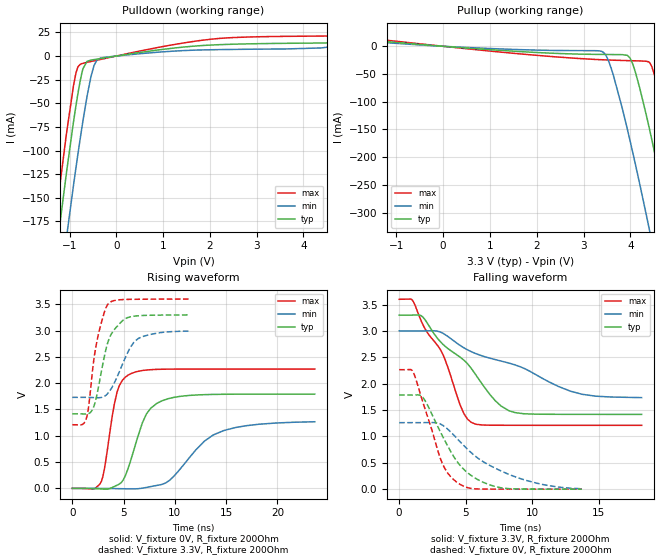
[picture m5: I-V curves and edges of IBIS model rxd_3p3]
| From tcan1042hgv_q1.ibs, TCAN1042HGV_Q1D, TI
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|   rxd_3p3 Model
[Model]   rxd_3p3
Model_type   Output
Polarity   Non-Inverting
Vmeas = 1.65
Vref = 0
Cref = 2pF
Rref = 350
|   typ   min   max
|   (nom PVT)   (fast PVT)   (slow PVT)
C_comp   2.461e-12   2.233e-12   2.954e-12
| Where nom  PVT is Nominal Process, 3.3V, 27C
|   Fast PVT is Strong Process,  3.6V, -55C
|   Slow PVT is Weak Process,   3V, 150C
[Voltage Range]   3.3   3   3.6
|Junction Temperature
[Temperature Range]   27   150   -55
[Pullup Reference]   3.3   3   3.6
[Pulldown Reference]   0   0   0
[Power Clamp Reference]   3.3   3   3.6
[GND Clamp Reference]   0   0   0
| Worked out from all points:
|   slope of the pulldown table from 0 to 0.495 V, typ, clamps not added: 133 ohm
|   slope of the pullup table from 0 to 0.495 V, typ, clamps not added: 158 ohm
|   falling waveform, V_fixture 3.3V, R_fixture 200Ohm: 20-80 % time 4.13ns typ, 7.18ns min, 2.68ns max; typ from 3.3 V to 1.42 V
|   rising waveform, V_fixture 0V, R_fixture 200Ohm: 20-80 % time 1.9ns typ, 3.72ns min, 1.14ns max; typ from 0 V to 1.79 V
|   rising waveform, V_fixture 3.3V, R_fixture 200Ohm: 20-80 % time 1.35ns typ, 1.83ns min, 1.12ns max; typ from 1.42 V to 3.3 V
|   falling waveform, V_fixture 0V, R_fixture 200Ohm: 20-80 % time 2.49ns typ, 4.32ns min, 1.73ns max; typ from 1.78 V to 0.001 V
[Pulldown]
|   Voltage   I(typ)   I(min)   I(max)
-3.3V     -1.124A    -1.169A    -1.104A
-1.392V   -254.1mA   -321.8mA   -214.6mA
-1.212V   -180.6mA   -249.2mA   -139.4mA
-1.062V   -122.4mA   -191.1mA   -81.02mA
-870mV    -54.95mA   -120.9mA   -19.69mA
-736.8mV  -18.03mA   -76.19mA   -8.057mA
-621.6mV  -5.53mA    -41.64mA   -6.593mA
-477mV    -3.737mA   -10.14mA   -5.058mA
-330mV    -2.573mA   -1.991mA   -3.502mA
2.16V     11.97mA    6.79mA     18.48mA
5.148V    14.26mA    13.31mA    21.37mA
6.6V      26.42mA    22.89mA    28.28mA
[Pullup]
|   Voltage   I(typ)   I(min)   I(max)
-3.3V     23.03mA    18.14mA    29.89mA
3.393V    -14.72mA   -9.431mA   -24.31mA
3.486V    -14.8mA    -17.71mA   -24.65mA
3.623V    -14.91mA   -48.3mA    -25.08mA
3.99V     -20.67mA   -169mA     -25.98mA
4.112V    -47.98mA   -214.5mA   -26.24mA
4.39V     -142.3mA   -324mA     -28.08mA
4.559V    -207.8mA   -393.9mA   -64.25mA
4.843V    -324.7mA   -515.2mA   -169.6mA
5.062V    -418.4mA   -610.8mA   -260.7mA
5.264V    -507mA     -700.4mA   -348.4mA
6.6V      -1.126A    -1.309A    -962mA
[Ramp]
R_load = 200
|   typ   min   max
dV/dt_r   1.07557/1.89697e-09  0.762875/3.74775e-09   1.36141/1.14474e-09
dV/dt_f   1.1294/4.13384e-09   0.761627/7.21056e-09   1.43384/2.67634e-09
[Falling Waveform]
V_fixture = 3.3V
V_fixture_min = 3V
V_fixture_max = 3.6V
R_fixture = 200Ohm
|   Time   V(typ)   V(min)   V(max)
0s        3.3V       3V         3.6V
1.078ns   3.301V     3V         3.551V
1.786ns   3.262V     3V         3.12V
3.27ns    2.752V     2.959V     2.565V
4.574ns   2.504V     2.728V     1.603V
5.429ns   2.287V     2.607V     1.266V
7.232ns   1.676V     2.457V     1.212V
8.727ns   1.451V     2.355V     1.211V
13.74ns   1.419V     1.8V       1.211V
18.23ns   1.418V     1.736V     1.21V
[Rising Waveform]
V_fixture = 0V
V_fixture_min = 0V
V_fixture_max = 0V
R_fixture = 200Ohm
|   Time   V(typ)   V(min)   V(max)
0s        67.61pV    49.82nV    41.37pV
2.723ns   -9.335mV   -270.6uV   90.03mV
3.129ns   -13.85mV   -1.243mV   366.2mV
4.361ns   59.96mV    -5.5mV     1.826V
4.97ns    160.6mV    -7.461mV   2.073V
5.763ns   575.3mV    -9.949mV   2.186V
7.232ns   1.417V     17.7mV     2.25V
8.727ns   1.664V     75.33mV    2.265V
14.78ns   1.789V     1.1V       2.269V
23.64ns   1.793V     1.267V     2.269V
[Rising Waveform]
V_fixture = 3.3V
V_fixture_min = 3V
V_fixture_max = 3.6V
R_fixture = 200Ohm
|   Time   V(typ)   V(min)   V(max)
0s        1.418V     1.731V     1.21V
1.336ns   1.413V     1.731V     1.309V
1.558ns   1.42V      1.73V      1.502V
1.933ns   1.484V     1.728V     2.166V
2.48ns    1.852V     1.723V     2.872V
3.129ns   2.51V      1.752V     3.35V
3.633ns   2.866V     1.847V     3.534V
4.97ns    3.2V       2.395V     3.591V
6.447ns   3.282V     2.851V     3.596V
11.44ns   3.299V     2.991V     3.6V
[Falling Waveform]
V_fixture = 0V
V_fixture_min = 0V
V_fixture_max = 0V
R_fixture = 200Ohm
|   Time   V(typ)   V(min)   V(max)
0s        1.785V     1.261V     2.265V
995.3ps   1.785V     1.261V     2.245V
1.786ns   1.739V     1.262V     1.647V
3.27ns    1.002V     1.212V     475.2mV
3.857ns   723.9mV    1.089V     241mV
4.574ns   454.6mV    901.7mV    92.05mV
5.919ns   180.3mV    589.5mV    4.289mV
7.649ns   27.11mV    346.9mV    949.4uV
10.73ns   1.183mV    92.08mV    371.3uV
13.74ns   523.8uV    8.027mV    203.3uV
